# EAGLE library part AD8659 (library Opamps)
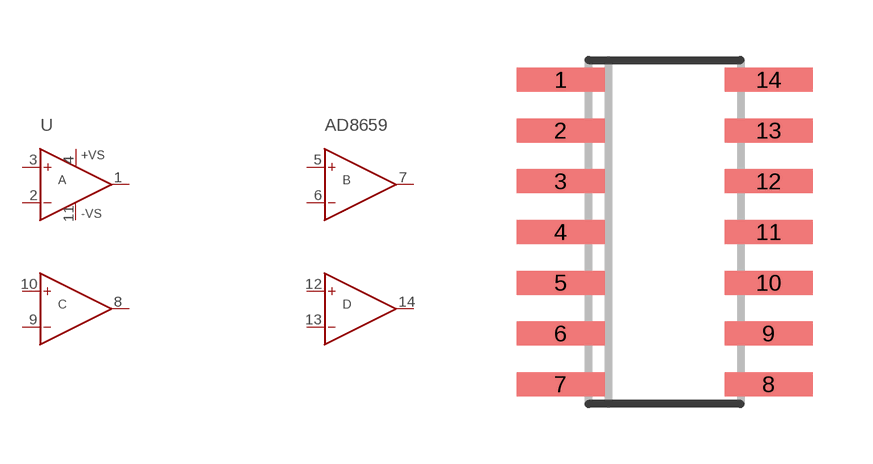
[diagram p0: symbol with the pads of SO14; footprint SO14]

Designator prefix U

## AD8659  [SO14]
1  OUTA  out
2  -INA  in
3  +INA  in
4  +VS  in
5  +INB  in
6  -INB  in
7  OUTB  out
8  OUTC  out
9  -INC  in
10  +INC  in
11  -VS  in
12  +IND  in
13  -IND  in
14  OUTD  out

## Footprint SO14 (pad centres in mm)
smd 2.2 x 0.6: 1 -2.6,3.81; 2 -2.6,2.54; 3 -2.6,1.27; 4 -2.6,0; 5 -2.6,-1.27; 6 -2.6,-2.54; 7 -2.6,-3.81; 8 2.6,-3.81; 9 2.6,-2.54; 10 2.6,-1.27; 11 2.6,0; 12 2.6,1.27; 13 2.6,2.54; 14 2.6,3.81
